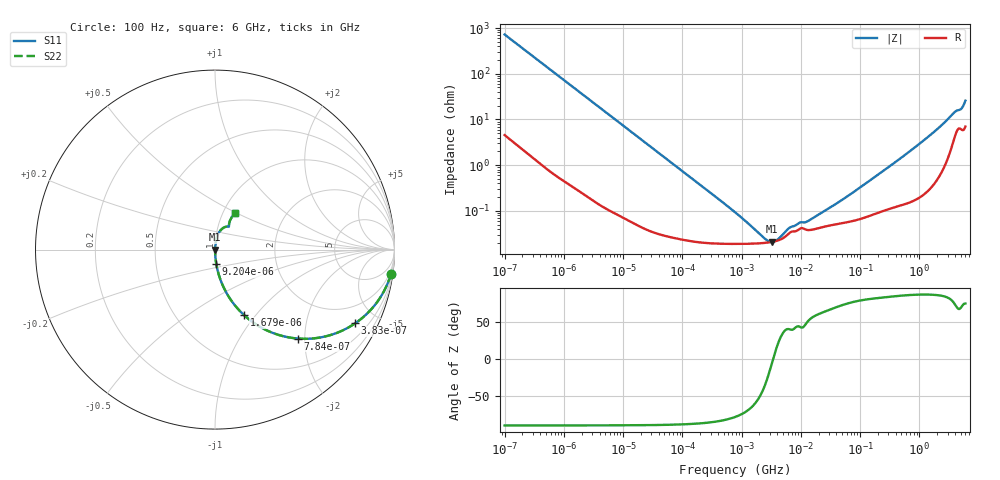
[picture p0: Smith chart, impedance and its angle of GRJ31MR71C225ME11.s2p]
!Murata Part Number: GRJ31MR71C225ME11
!These Parameters are Measured in Series Mode Connection
!Data Generated on Jun 19, 2026
!  o--ll--o
!Port1  Port2
!  o------o
!Operation Temp=25[degC], DC Bias Voltage=0[V]
!Freq. Start=100[Hz] Stop=6[GHz] 401[Steps]
# Hz S RI R 50
!Freq.(Hz) S11(Real) S11(Imag) S21(Real) S21(Imag) S12(Real) S12(Imag) S22(Real) S22(Imag)
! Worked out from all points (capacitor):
!   401 points, 100 Hz to 6 GHz, reference 50 ohm
!   read as one part in series: C = 2.2 uF near 109 Hz
!   lowest |Z| = 21 mohm at 3.246 MHz (marker M1)
!   series resonance near 3.416 MHz, so ESL is about 990 pH
!   S11 on the Smith chart (normalised r, x): 100 Hz: 1, -14; 383 Hz: 1.02, -3.79; 784 Hz: 1.01, -1.86; 1.679 kHz: 1.01, -0.87; 9.204 kHz: 1.00, -0.16; 6 GHz: 1.14, +0.49
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100  0.9804 -0.1356  0.0196 0.1356  0.0196 0.1356  0.9804 -0.1356
205  0.9248 -0.2608  0.0752 0.2608  0.0752 0.2608  0.9248 -0.2608
383  0.781 -0.4107  0.219 0.4107  0.219 0.4107  0.781 -0.4107
573  0.6162 -0.4834  0.3838 0.4834  0.3838 0.4834  0.6162 -0.4834
784  0.4631 -0.4957  0.5369 0.4957  0.5369 0.4957  0.4631 -0.4957
1679  0.1607 -0.3639  0.8393 0.3639  0.8393 0.3639  0.1607 -0.3639
2008  0.1186 -0.3199  0.8814 0.3199  0.8814 0.3199  0.1186 -0.3199
3759  0.0378 -0.1872  0.9622 0.1872  0.9622 0.1872  0.0378 -0.1872
9204  0.00707 -0.0793  0.9929 0.0793  0.9929 0.0793  0.00707 -0.0793
40335  0.000644 -0.0183  0.9994 0.0183  0.9994 0.0183  0.000644 -0.0183
774597  0.00019 -0.000915  0.9998 0.000915  0.9998 0.000915  0.00019 -0.000915
2372521  0.000198 -0.000164  0.9998 0.000164  0.9998 0.000164  0.000198 -0.000164
3245845  0.000209 -2.25e-05  0.9998 2.25e-05  0.9998 2.25e-05  0.000209 -2.25e-05
4060267  0.000224 7.71e-05  0.9998 -7.71e-05  0.9998 -7.71e-05  0.000224 7.71e-05
6644369  0.000339 0.000276  0.9997 -0.000276  0.9997 -0.000276  0.000339 0.000276
1.555665e7  0.000387 0.000561  0.9996 -0.000561  0.9996 -0.000561  0.000387 0.000561
5.449875e7  0.000551 0.00179  0.9994 -0.00179  0.9994 -0.00179  0.000551 0.00179
3.124326e8  0.00119 0.00925  0.9988 -0.00925  0.9988 -0.00925  0.00119 0.00925
1.873145e9  0.00734 0.0559  0.9927 -0.0559  0.9927 -0.0559  0.00734 0.0559
3.8344e9  0.0507 0.1236  0.9493 -0.1236  0.9493 -0.1236  0.0507 0.1236
5.016141e9  0.0778 0.1351  0.9222 -0.1351  0.9222 -0.1351  0.0778 0.1351
6e9  0.1128 0.205  0.8872 -0.205  0.8872 -0.205  0.1128 0.205
